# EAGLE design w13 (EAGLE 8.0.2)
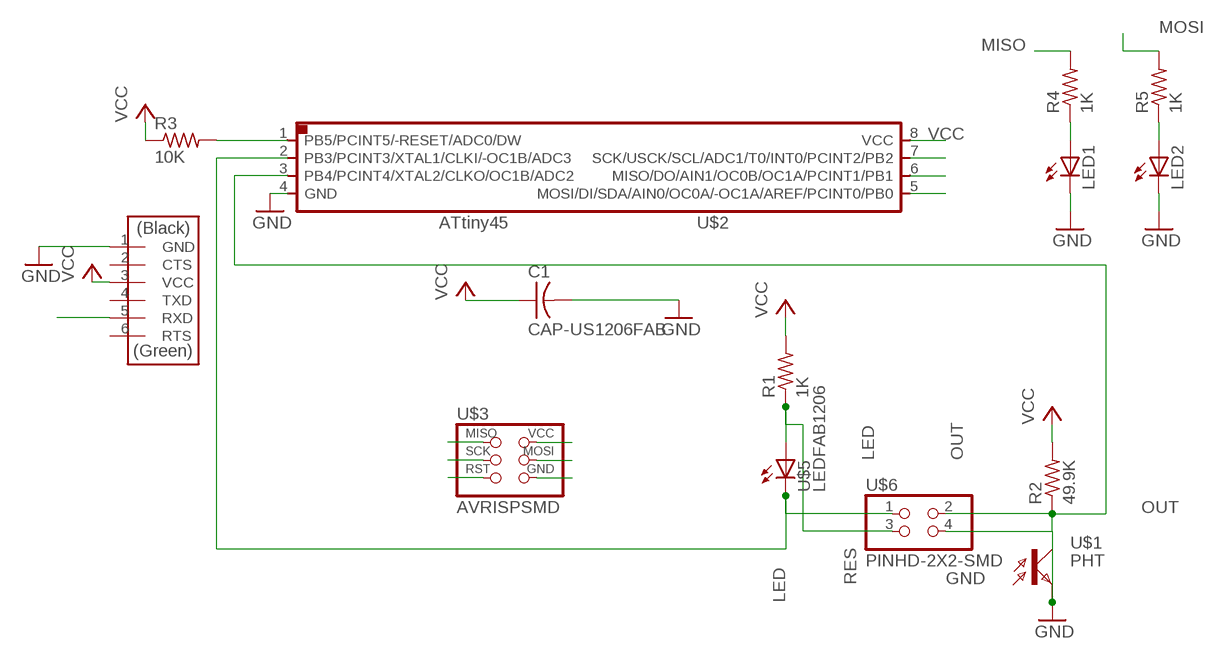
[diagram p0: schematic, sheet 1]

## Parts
C1  CAP-US1206FAB  [C1206FAB]
LED1  LED3MM  [LED3MM]
LED2  LED3MM  [LED3MM]
R1  1K  RES-US1206FAB  [R1206FAB]
R2  49.9K  RES-US1206FAB  [R1206FAB]
R3  10K  RES-US1206FAB  [R1206FAB]
R4  1K  RES-US1206FAB  [R1206FAB]
R5  1K  RES-US1206FAB  [R1206FAB]
U$1  PHT  PHOTOTRANSISTOR-NPN1206  [OP1206]
U$2  ATTINY45SI  [SOIC8]
U$3  AVRISPSMD  [2X03SMD]
U$4  FTDI-SMD-HEADER  [1X06SMD]
U$5  LEDFAB1206  [LED1206FAB]
U$6  PINHD-2X2-SMD  [2X02SMD]

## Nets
GND: C1.2 LED1.K(C) LED2.K(C) U$1.EMITTER(E) U$2.4(GND) U$3.6(GND) U$4.1(GND) U$6.4
LED: U$2.2(PB3/PCINT3/XTAL1/CLKI/-OC1B/ADC3) U$5.2(C) U$6.1
MISO: R4.2 U$2.6(MISO/DO/AIN1/OC0B/OC1A/PCINT1/PB1) U$3.1(MISO)
MOSI: R5.2 U$2.5(MOSI/DI/SDA/AIN0/OC0A/-OC1A/AREF/PCINT0/PB0) U$3.4(MOSI)
N$2: LED1.A R4.1
N$3: LED2.A R5.1
OUT: R2.1 U$1.COLLECTOR(C) U$2.3(PB4/PCINT4/XTAL2/CLKO/OC1B/ADC2) U$6.2
RES: R1.1 U$5.1(A) U$6.3
RST: R3.2 U$2.1(PB5/PCINT5/-RESET/ADC0/DW) U$3.5(RST)
SCK: U$2.7(SCK/USCK/SCL/ADC1/T0/INT0/PCINT2/PB2) U$3.3(SCK) U$4.5(RXD)
VCC: C1.1 R1.2 R2.2 R3.1 U$2.8(VCC) U$3.2(VCC) U$4.3(VCC)
Unconnected: U$4.2(CTS) U$4.4(TXD) U$4.6(RTS)

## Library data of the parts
C1 = fab:CAP-US
LED1 LED2 = led:LED: LED
R1-R5 = fab:RES-US: Resistor (US Symbol)
U$1 = fab:PHOTOTRANSISTOR-NPN
U$2 = fab:ATTINY45
U$3 = fab:AVRISP
U$4 = fab:FTDI-SMD-HEADER
U$5 = fab:LED: LED
U$6 = fab:PINHD-2X2-SMD

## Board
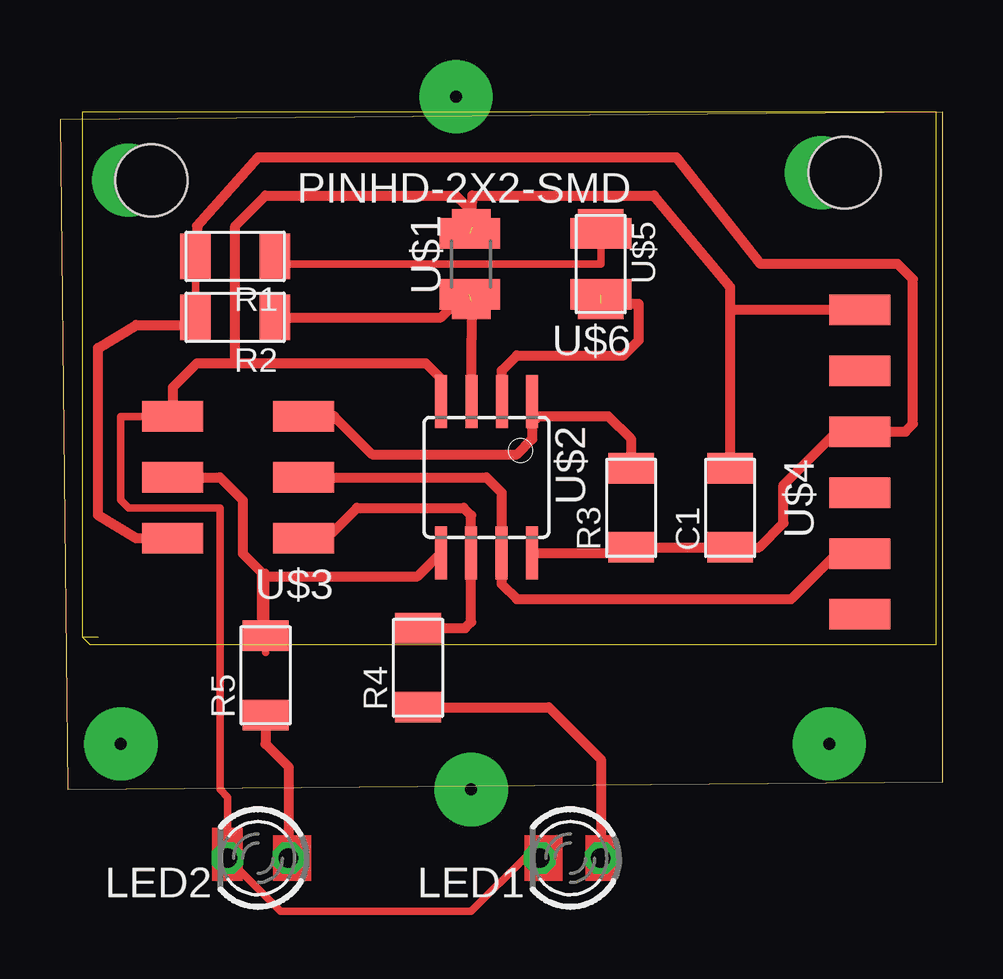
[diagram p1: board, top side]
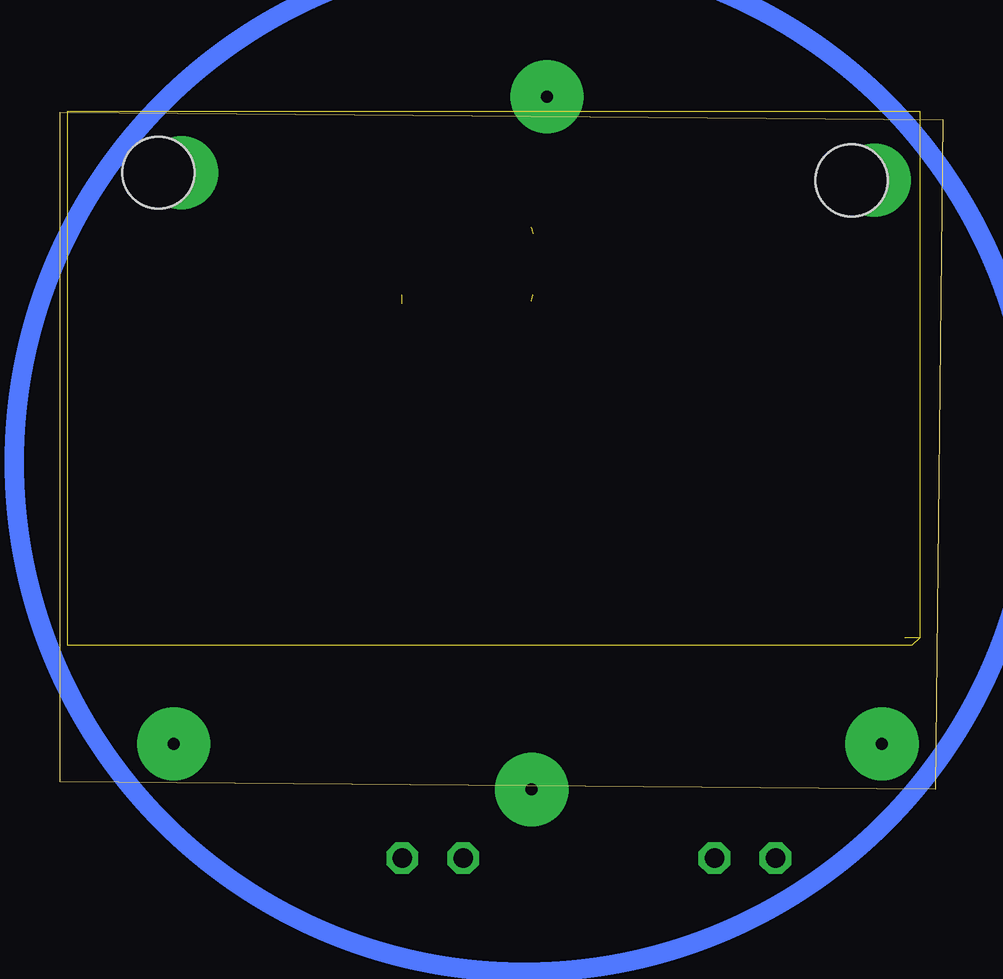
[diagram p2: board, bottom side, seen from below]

Size 36.81 x 28.24 mm. Coordinates in mm from the lower left corner, seen from the top.
Outline: 0.32,0 36.81,0.32 36.81,28.25 0,27.93 0.32,0
Copper layers (1*16): Top 0.035mm / dielectric 1.5mm / Bottom 0.035mm
Design rules "default": minimum track width 10mil, minimum drill 24mil, track to track 8mil, track to pad 8mil, pad to pad 8mil, via to via 8mil, smd to smd 8mil, copper to edge 40mil, drill to drill 8mil, minimum pad ring 10mil, minimum via ring 8mil, stop-mask expansion 4mil, vias tented up to drill 0mil, thermal gap 10mil
Holes 3 mm at 3.81,25.4 32.7,25.72

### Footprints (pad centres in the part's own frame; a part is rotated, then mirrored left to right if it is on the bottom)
C1206FAB = smd 1.27 x 1.905: 1 -1.651,0; 2 1.651,0
LED3MM = drill 0.813 octagon: A -1.27,0; K 1.27,0
R1206FAB = smd 1.27 x 1.905: 1 -1.651,0; 2 1.651,0
OP1206 = smd 1.5 x 1.6: COLLECTOR -1.55,0; EMITTER 1.55,0
SOIC8 = smd 0.5 x 2.2: 1 -1.905,-3.154; 2 -0.645,-3.154; 3 0.625,-3.154; 4 1.895,-3.154; 5 1.905,3.154; 6 0.635,3.154; 7 -0.635,3.154; 8 -1.905,3.154
2X03SMD = smd 2.54 x 1.27: 1 -2.54,2.54; 2 2.92,2.54; 3 -2.54,0; 4 2.92,0; 5 -2.54,-2.54; 6 2.92,-2.54
1X06SMD = smd 2.54 x 1.27: 1 0,6.35; 2 0,3.81; 3 0,1.27; 4 0,-1.27; 5 0,-3.81; 6 0,-6.35
LED1206FAB = smd 1.27 x 1.905: 1 -1.651,0; 2 1.651,0
2X02SMD = smd 2.54 x 1.27: 1 -2.54,1.27; 2 2.92,1.27; 3 -2.54,-1.27; 4 2.92,-1.27

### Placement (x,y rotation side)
C1  27.94,11.75 90 top
LED1  21.27,-2.86 180 top
LED2  8.26,-2.86 180 top
R1  7.3,22.23 180 top
R2  7.3,19.68 180 top
R3  23.81,11.75 90 top
R4  14.92,5.08 90 top
R5  8.57,4.76 90 top
U$1  17.14,21.91 90 top
U$2  17.78,13.02 180 top
U$3  7.62,13.02 180 top
U$4  33.34,13.65 0 top
U$5  22.54,21.91 270 top
U$6  20,21.91 180 top

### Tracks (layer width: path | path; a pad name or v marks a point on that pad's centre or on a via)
GND  (1 unrouted)
  Top 0.305: 15.88,17.15 15.88,16.18 U$2.4 | 17.14,24.13 U$1.EMITTER 17.18,23.46 17.18,24.76 | U$3.6 2.54,15.56 2.54,12.07 2.86,11.75 6.67,11.75 6.67,0 6.99,-0.32 LED2.K 9.21,-5.08 17.14,-5.08 19.37,-2.86 LED1.K
  Top 0.406: U$3.6 4.7,16.76 5.71,17.78 7.3,17.78 | 7.3,17.78 15.24,17.78 15.88,17.15 | 7.3,17.78 7.3,23.5 8.57,24.76 16.51,24.76 17.14,24.13 | C1.2 27.94,20 | 27.94,20 27.94,20.95 24.77,24.76 17.18,24.76 U$1.EMITTER | 27.94,20 U$4.1
LED  (1 unrouted)
  Top 0.305: U$5.2 23.18,20.26
  Top 0.406: U$2.2 18.43,17.47 19.05,18.1 23.5,18.1 24.13,18.73 24.13,20.26 23.18,20.26 U$5.2
MISO
  Top 0.305: U$3.1 11.11,10.48
  Top 0.406: 11.11,10.48 12.38,11.75 16.83,11.75 17.14,11.43 U$2.6 17.14,6.99 16.89,6.73 R4.2
MOSI
  Top 0.305: 8.41,9.05 8.57,9.05 8.57,6.99 R5.2 | R5.2 8.57,5.71 R5.2
  Top 0.406: U$3.4 6.67,13.02 7.62,12.07 7.62,9.84 8.41,9.05 | 8.41,9.05 8.57,8.89 14.9,8.89 U$2.5 | 8.41,9.05 8.41,7.14 8.57,6.99
N$1  (6 unrouted)
N$2
  Top 0.406: R4.1 20.38,3.43 22.54,1.27 LED1.A
N$3
  Top 0.406: R5.1 8.57,1.9 9.53,0.95 LED2.A
N$4  (via drill 0.5 pad 3.05)
  other vias: 2.86,25.4
N$5  (via drill 0.5 pad 3.05)
  other vias: 31.75,25.72
N$6  (via drill 0.5 pad 3.05)
  other vias: 2.54,1.9
N$7  (via drill 0.5 pad 3.05)
  other vias: 32.07,1.9
N$8  (via drill 0.5 pad 3.05)
  other vias: 16.51,28.89
N$9  (via drill 0.5 pad 3.05)
  other vias: 17.14,0
OUT  (1 unrouted)
  Top 0.305: 16.51,20.32 17.11,20.32 U$1.COLLECTOR 17.15,19.69
  Top 0.406: U$2.3 17.16,18.76 17.15,19.69 U$1.COLLECTOR | R2.1 15.88,19.68 16.51,20.32
RES
  Top 0.305: 9.27,21.91 R1.1 8.95,21.91 22.54,21.91 U$6.3 | U$6.3 U$5.1 U$6.3
RST
  Top 0.305: U$3.5 11.43,15.56 | U$2.1 19.68,15.24 20,15.56
  Top 0.406: 11.43,15.56 13.02,13.97 19.05,13.97 19.68,14.6 19.68,15.24 | R3.2 23.81,14.6 22.86,15.56 20,15.56
SCK
  Top 0.305: 32.38,9.84 U$4.5
  Top 0.406: U$3.3 17.78,13.02 18.41,12.38 U$2.7 18.41,8.57 19.05,7.94 30.48,7.94 32.38,9.84
VCC
  Top 0.305: 23.58,9.86 R3.1 | 5.65,21.59 R2.2 5.33,19.37 | 5.65,21.59 R1.2 | 32.38,14.92 U$4.3 | 5.71,21.65 5.65,21.59
  Top 0.406: R3.1 C1.1 29.15,10.1 30.16,11.11 30.16,12.7 32.38,14.92 | U$2.8 23.58,9.86 | U$3.2 3.18,10.48 1.59,11.43 1.59,18.42 3.18,19.37 5.33,19.37 | U$4.3 35.24,14.92 35.56,15.24 35.56,21.27 34.92,21.91 29.21,21.91 25.72,26.35 8.26,26.35 5.71,23.5 5.71,21.65
(copper drawn outside any net)
  shapes: Bottom circle x1, Top area x5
